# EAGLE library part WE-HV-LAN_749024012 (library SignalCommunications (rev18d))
WE-LAN HV LAN-Transformer Characteristics: •Compliant with IEEE802.3 and 802.3af standards •Operating temperature: 0 °C to +70 °C •SMD •4 kV Hipot test Applications: •Ethernet •Compliant with most IC's for Ethernet applications like Intel, AMD, Conexant, Realtek, etc. •Hub, Router, Switches, medical applications Details see: http://katalog.we-online.de/en/pbs/WE-LAN/749024012? Updated by Dan Xu 2014-07-08 2014 (C) Würth Elektronik
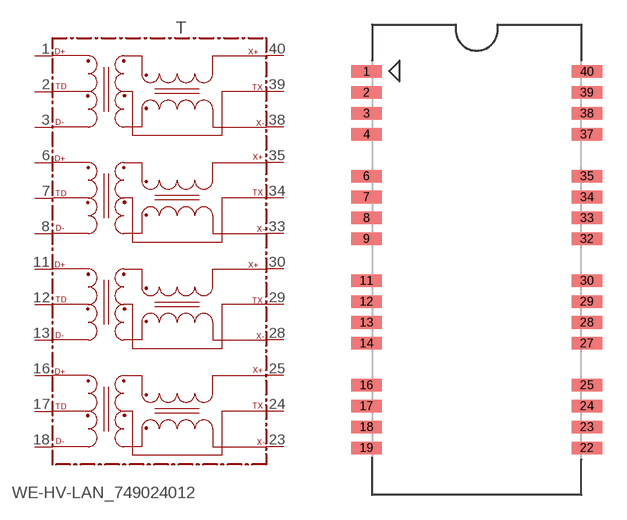
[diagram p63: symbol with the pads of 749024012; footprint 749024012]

Designator prefix T

## WE-HV-LAN_749024012  [749024012]
1  D+
2  TD
3  D-
6  D1+
7  TD1
8  D1-
11  D2+
12  TD2
13  D2-
16  D3+
17  TD3
18  D3-
23  X3-
24  TX3
25  X3+
28  X2-
29  TX2
30  X2+
33  X1-
34  TX1
35  X1+
38  X-
39  TX
40  X+

## Footprint 749024012 (pad centres in mm)
MAX Height=12.70 mm
smd 1.86 x 0.76: 1 -6.69,11.43; 2 -6.69,10.16; 3 -6.69,8.89; 4 -6.69,7.62; 6 -6.69,5.08; 7 -6.69,3.81; 8 -6.69,2.54; 9 -6.69,1.27; 11 -6.69,-1.27; 12 -6.69,-2.54; 13 -6.69,-3.81; 14 -6.69,-5.08; 16 -6.69,-7.62; 17 -6.69,-8.89; 18 -6.69,-10.16; 19 -6.69,-11.43; 22 6.69,-11.43; 23 6.69,-10.16; 24 6.69,-8.89; 25 6.69,-7.62; 27 6.69,-5.08; 28 6.69,-3.81; 29 6.69,-2.54; 30 6.69,-1.27; 32 6.69,1.27; 33 6.69,2.54; 34 6.69,3.81; 35 6.69,5.08; 37 6.69,7.62; 38 6.69,8.89; 39 6.69,10.16; 40 6.69,11.43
